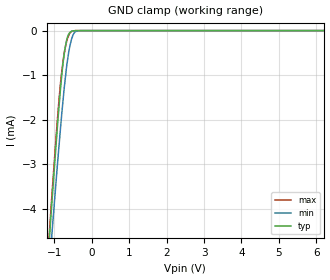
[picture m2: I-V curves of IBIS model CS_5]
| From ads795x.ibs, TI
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|   Input CS model 5V
[Model]   CS_5
Model_type   Input
|Signals   CS
Enable   Active-Low
Vinl = 0.8
Vinh = 3.5
|   typ   min   max
C_comp   6.1532919e-13  6.8525286e-13   5.4770236e-13
[Voltage Range]   5   4.75   5.25
[Temperature Range]   27   125   -40
[Pullup Reference]   5   4.75   5.25
[Pulldown Reference]   0   0   0
[Power Clamp Reference]   5   4.75   5.25
[GND Clamp Reference]   0   0   0
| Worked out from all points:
|   GND clamp passes 1 mA (typ) near -0.80 V on its own axis
[GND Clamp]
|   Voltage   I(typ)   I(min)   I(max)
-5V       -55.07mA   -50.46mA   -60.71mA
-1.167V   -5.081mA   -5.675mA   -4.96mA
-1.113V   -4.42mA    -5.09mA    -4.287mA
-1.072V   -3.928mA   -4.64mA    -3.771mA
-1.032V   -3.457mA   -4.209mA   -3.306mA
-944.1mV  -2.444mA   -3.281mA   -2.279mA
-815.6mV  -1.119mA   -1.992mA   -1.015mA
-724.7mV  -444.9uA   -1.197mA   -455.9uA
-675.3mV  -224.8uA   -825.9uA   -251uA
-523.7mV  -9.12uA    -149.7uA   -14.75uA
-314.2mV  -601.4nA   -761.3nA   -1.034uA
9.985V    0A         0A         0A
[POWER Clamp]
|   No ESD cells to VDD
|   Voltage   I(typ)   I(min)   I(max)
-5V       0A         0A         0A
0V        0A         0A         0A
10V       0A         0A         0A
